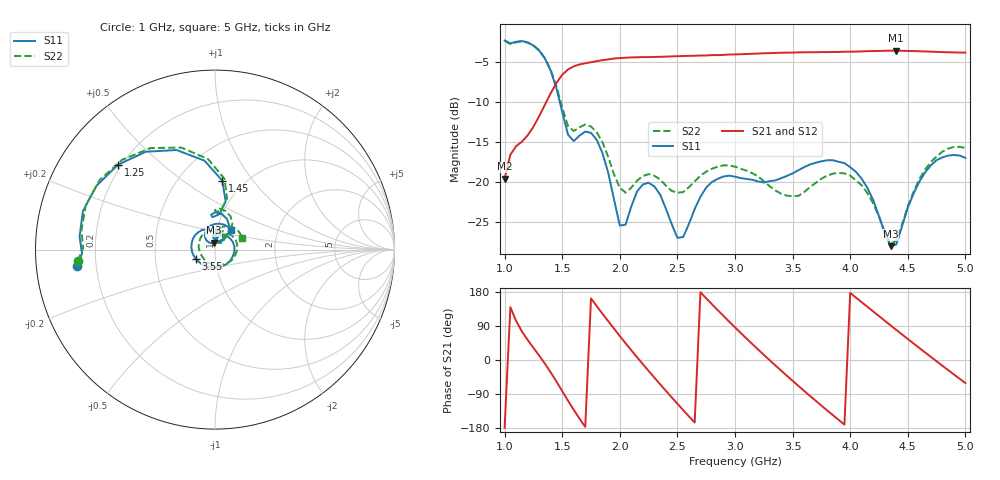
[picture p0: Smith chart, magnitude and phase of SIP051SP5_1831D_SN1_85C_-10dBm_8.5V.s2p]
# GHz  S  dB  R  50
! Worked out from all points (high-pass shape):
!   81 points, 1 GHz to 5 GHz, reference 50 ohm
!   highest |S21| = -3.52 dB at 4.4 GHz (marker M1); lowest = -19.6 dB at 1 GHz (marker M2)
!   |S21| within 3 dB of the highest: 1.503 GHz to end of sweep
!   lowest |S11| = -28.0 dB at 4.35 GHz (marker M3), VSWR 1.08, Z = 49 + j3.8 ohm
!   |S11| at or under -10 dB: 1.48 GHz to end of sweep
!   |S22| runs from -27.7 to -2.3 dB; largest |S21 - S12| = 0.0021
!   S11 on the Smith chart (normalised r, x): 1 GHz: 0.13, -0.06; 1.25 GHz: 0.19, +0.36; 1.45 GHz: 0.79, +0.72; 3.55 GHz: 0.80, -0.08; 5 GHz: 1.16, +0.26
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1  -2.24 -173.1  -19.57 -179.0  -19.59 -179.2  -2.29 -175.2
1.25  -2.88 138.8  -13.07 32.2  -13.06 32.2  -2.86 135.9
1.45  -8.25 84.1  -7.56 -56.8  -7.55 -56.8  -8.00 82.4
1.55  -14.05 82.9  -5.89 -107.2  -5.87 -107.2  -12.97 80.9
1.7  -13.67 90.1  -5.10 -176.5  -5.09 -176.4  -12.79 83.9
1.85  -16.40 57.7  -4.71 121.9  -4.71 121.9  -15.04 56.9
1.95  -22.19 48.5  -4.51 82.6  -4.51 82.6  -19.06 50.0
2.05  -25.35 89.7  -4.41 44.4  -4.40 44.4  -21.33 67.4
2.15  -21.18 95.0  -4.35 7.2  -4.34 7.2  -19.84 74.1
2.35  -21.57 57.1  -4.29 -63.9  -4.27 -64.0  -19.67 55.5
2.5  -27.00 58.1  -4.21 -115.4  -4.20 -115.4  -21.34 54.5
2.7  -21.85 72.3  -4.13 178.8  -4.12 178.9  -19.20 52.9
2.85  -19.60 36.4  -4.08 131.6  -4.07 131.6  -18.06 32.7
3  -19.33 -6.5  -3.99 86.1  -3.97 86.1  -18.07 6.6
3.3  -19.89 -95.0  -3.83 -0.3  -3.82 -0.3  -20.51 -62.2
3.55  -18.52 -154.2  -3.73 -68.2  -3.73 -68.3  -21.73 -153.2
3.7  -17.58 174.0  -3.72 -107.5  -3.71 -107.4  -20.11 153.8
4  -18.13 114.8  -3.65 177.1  -3.65 177.1  -19.19 78.8
4.35  -28.04 102.1  -3.52 91.6  -3.54 91.6  -27.74 62.3
4.4  -27.84 120.3  -3.52 79.4  -3.52 79.5  -27.38 78.8
4.7  -17.90 107.7  -3.64 8.2  -3.63 8.2  -17.49 72.2
5  -16.97 51.2  -3.77 -60.9  -3.76 -61.0  -15.73 22.3
